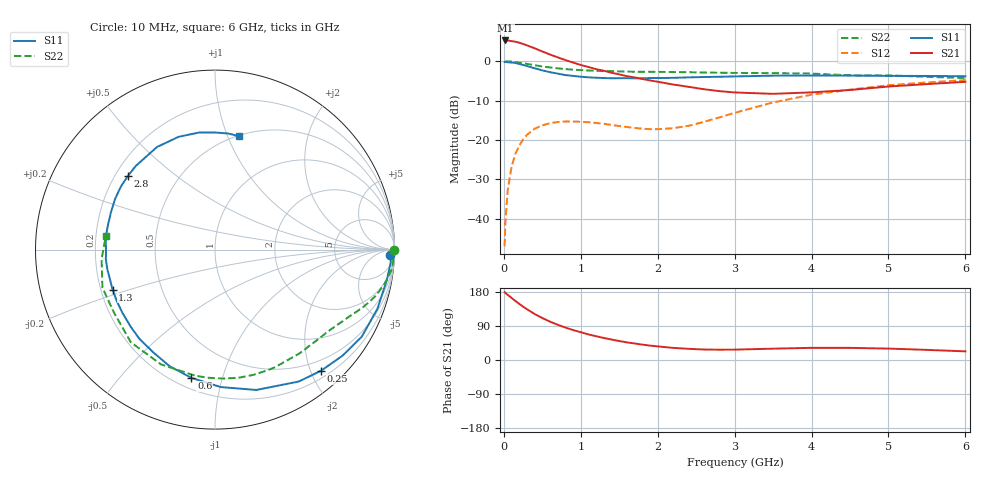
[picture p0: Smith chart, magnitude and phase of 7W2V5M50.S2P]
! Infineon Technologies  Discrete & RF Semiconductors
! BFS17W
! Si NPN RF Bipolar Junction Transistor in SOT323
! VCE = 2.5 V  IC = 0.5 mA
! Common Emitter S-Parameters:  August  1999
# GHz  S  MA  R  50
!  f  S11  S21  S12  S22
! GHz  MAG  ANG  MAG  ANG  MAG  ANG  MAG  ANG
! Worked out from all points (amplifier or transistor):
!   36 points, 10 MHz to 6 GHz, reference 50 ohm
!   highest |S21| = 5.3 dB at 20 MHz (marker M1)
!   |S21| within 3 dB of that: start of sweep to 526.1 MHz
!   unconditionally stable (mu >= 1): 1.181 GHz to end of sweep
!   at 250 MHz: K = 0.23, MSG = 12.1 dB, |S12| = -19.9 dB
!   at 1.4 GHz: K = 1.18, MAG = 4.1 dB, |S12| = -16.2 dB
!   at 6 GHz: K = 1.11, MAG = -2.2 dB, |S12| = -4.8 dB
!   S11 on the Smith chart (normalised r, x): 10 MHz: 29, -40; 250 MHz: 0.31, -2.17; 600 MHz: 0.26, -0.80; 1.3 GHz: 0.25, -0.18; 2.8 GHz: 0.25, +0.35; 6 GHz: 0.51, +1.10
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0.01  0.9765 -1.9  1.829 179.2  0.0045 86.9  0.9999 -0.1
0.02  0.9818 -4.2  1.837 177.0  0.0091 92.7  0.9868 -1.2
0.05  0.9721 -10.2  1.834 171.8  0.0228 84.7  0.9955 -3.2
0.1  0.9632 -20.0  1.803 164.0  0.0456 78.0  0.9914 -6.2
0.15  0.9509 -30.7  1.768 155.8  0.0666 71.5  0.9758 -9.1
0.25  0.897 -48.8  1.658 140.9  0.1015 60.4  0.9428 -14.3
0.3  0.8706 -57.6  1.591 134.1  0.1164 56.0  0.927 -16.6
0.4  0.8152 -73.6  1.463 121.4  0.1392 47.4  0.891 -20.6
0.5  0.7666 -87.6  1.331 110.8  0.1536 40.6  0.8591 -23.9
0.6  0.7266 -100.4  1.218 101.2  0.1637 35.0  0.8335 -26.8
0.8  0.6679 -121.0  1.036 85.6  0.172 27.0  0.7955 -32.4
1.1  0.6249 -145.5  0.845 67.5  0.1685 20.5  0.7635 -40.2
1.3  0.6127 -158.7  0.758 58.1  0.1612 19.3  0.7504 -45.9
1.6  0.6105 -174.9  0.646 46.4  0.1465 21.5  0.7394 -54.5
2.2  0.6161 160.2  0.507 32.0  0.1413 41.4  0.7301 -73.1
2.8  0.6356 139.7  0.418 27.2  0.1933 58.4  0.7153 -92.7
3.5  0.6566 119.5  0.386 29.9  0.3001 59.8  0.7068 -115.1
4  0.6603 107.9  0.403 32.1  0.3765 54.2  0.6976 -132.2
4.5  0.6583 97.7  0.432 32.0  0.4362 47.4  0.6635 -147.9
5  0.6525 90.0  0.478 30.1  0.4959 40.7  0.6621 -161.3
5.5  0.6509 83.5  0.513 26.7  0.5381 34.1  0.6342 -175.2
6  0.646 78.0  0.548 22.8  0.5765 28.1  0.6125 172.8
